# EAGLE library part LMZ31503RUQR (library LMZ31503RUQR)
Non-Isolated DC/DC Converters 3A Power Module w/ 4.5V-14.5V Input Source: Datasheet
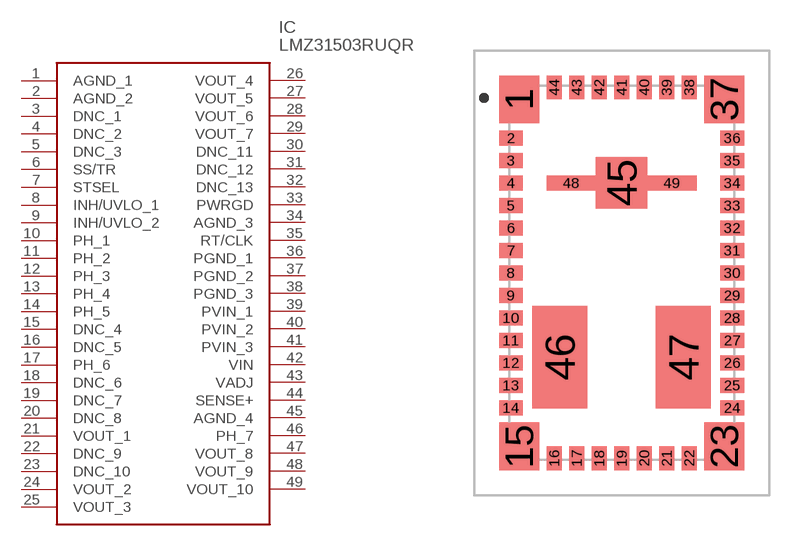
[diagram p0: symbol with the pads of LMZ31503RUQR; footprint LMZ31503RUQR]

Designator prefix IC

## LMZ31503RUQR (Description: Non-Isolated DC/DC Converters 3A Power Module w/ 4.5V-14.5V Input; Height: 2mm; Manufacturer_Name: Texas Instruments; Manufacturer_Part_Number: LMZ31503RUQR; Mouser_Part_Number: 595-LMZ31503RUQR; Mouser_Price-Stock: https://www.mouser.co.uk/ProductDetail/Texas-Instruments/LMZ31503RUQR?qs=Y1omCn8sZEXT19uo6SJdFA%3D%3D)  [LMZ31503RUQR]
1  AGND_1
2  AGND_2
3  DNC_1
4  DNC_2
5  DNC_3
6  SS/TR
7  STSEL
8  INH/UVLO_1
9  INH/UVLO_2
10  PH_1
11  PH_2
12  PH_3
13  PH_4
14  PH_5
15  DNC_4
16  DNC_5
17  PH_6
18  DNC_6
19  DNC_7
20  DNC_8
21  VOUT_1
22  DNC_9
23  DNC_10
24  VOUT_2
25  VOUT_3
26  VOUT_4
27  VOUT_5
28  VOUT_6
29  VOUT_7
30  DNC_11
31  DNC_12
32  DNC_13
33  PWRGD
34  AGND_3
35  RT/CLK
36  PGND_1
37  PGND_2
38  PGND_3
39  PVIN_1
40  PVIN_2
41  PVIN_3
42  VIN
43  VADJ
44  SENSE+
45  AGND_4
46  PH_7
47  VOUT_8
48  VOUT_9
49  VOUT_10

## Footprint LMZ31503RUQR (pad centres in mm)
RUQ0047A
smd 1.6 x 1.9: 1 -4.1,6.95; 15 -4.1,-6.95; 23 4.1,-6.95; 37 4.1,6.95
smd 0.95 x 0.6: 2 -4.425,5.4; 3 -4.425,4.5; 4 -4.425,3.6; 5 -4.425,2.7; 6 -4.425,1.8; 7 -4.425,0.9; 8 -4.425,0; 9 -4.425,-0.9; 10 -4.425,-1.8; 11 -4.425,-2.7; 12 -4.425,-3.6; 13 -4.425,-4.5; 14 -4.425,-5.4; 24 4.425,-5.4; 25 4.425,-4.5; 26 4.425,-3.6; 27 4.425,-2.7; 28 4.425,-1.8; 29 4.425,-0.9; 30 4.425,0; 31 4.425,0.9; 32 4.425,1.8; 33 4.425,2.7; 34 4.425,3.6; 35 4.425,4.5; 36 4.425,5.4
smd 0.6 x 0.95: 16 -2.7,-7.425; 17 -1.8,-7.425; 18 -0.9,-7.425; 19 0,-7.425; 20 0.9,-7.425; 21 1.8,-7.425; 22 2.7,-7.425; 38 2.7,7.425; 39 1.8,7.425; 40 0.9,7.425; 41 0,7.425; 42 -0.9,7.425; 43 -1.8,7.425; 44 -2.7,7.425
smd 2.05 x 2.05: 45 0,3.6
smd 2.2 x 4.1: 46 -2.475,-3.375; 47 2.475,-3.375
smd 1.975 x 0.6: 48 -2.012,3.6; 49 2.013,3.6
